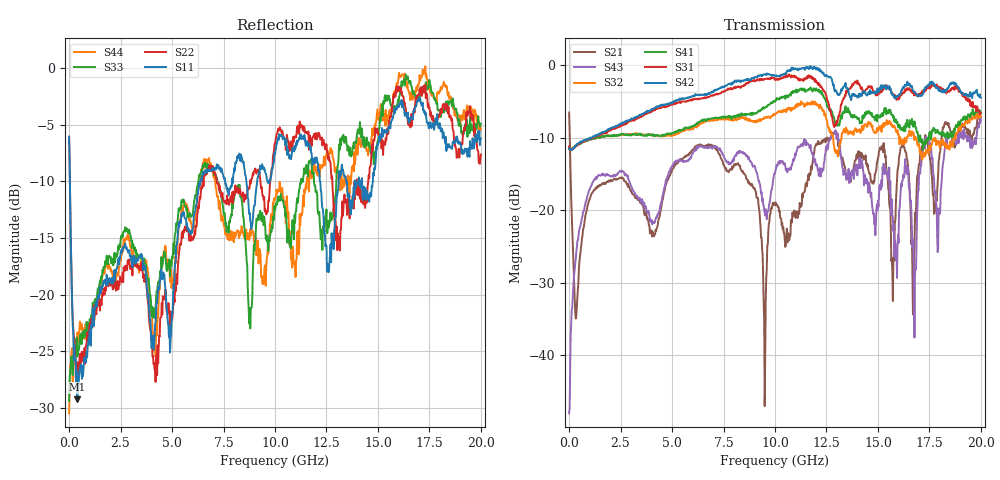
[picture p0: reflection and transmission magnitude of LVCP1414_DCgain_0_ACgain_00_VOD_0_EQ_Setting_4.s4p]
!Agilent Technologies,N5230A,MY46400459,A.07.50.48
!Agilent N5230A: A.07.50.48
!Date: Tuesday, April 17, 2012 18:34:43
!Correction: S11(Full 4 Port(1,2,3,4))
!S12(Full 4 Port(1,2,3,4))
!S13(Full 4 Port(1,2,3,4))
!S14(Full 4 Port(1,2,3,4))
!S21(Full 4 Port(1,2,3,4))
!S22(Full 4 Port(1,2,3,4))
!S23(Full 4 Port(1,2,3,4))
!S24(Full 4 Port(1,2,3,4))
!S31(Full 4 Port(1,2,3,4))
!S32(Full 4 Port(1,2,3,4))
!S33(Full 4 Port(1,2,3,4))
!S34(Full 4 Port(1,2,3,4))
!S41(Full 4 Port(1,2,3,4))
!S42(Full 4 Port(1,2,3,4))
!S43(Full 4 Port(1,2,3,4))
!S44(Full 4 Port(1,2,3,4))
!S4P File: Measurements: <S11,S12,S13,S14>,
!<S21,S22,S23,S24>,
!<S31,S32,S33,S34>,
!<S41,S42,S43,S44>:
# Hz S  dB  R 50
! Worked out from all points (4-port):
!   801 points, 300 kHz to 20 GHz, reference 50 ohm
!   strongest paths, dB at 300 kHz, 5 GHz, 10 GHz, 15 GHz, 20 GHz:
!     S42: -11.5, -5.1, -1.5, -3.4, -4.5
!     S31: -11.2, -5.4, -2.0, -4.1, -6.6
!     S41: -11.3, -9.3, -5.0, -7.0, -6.5
!     S32: -11.4, -9.7, -6.7, -9.0, -7.1
!     S43: -48.1, -13.9, -14.9, -18.7, -7.6
!     S21: -6.5, -14.4, -19.3, -12.8, -7.1
!   lowest |S11| = -29.2 dB at 400.3 MHz (marker M1), VSWR 1.07, Z = 53.2 + j1.51 ohm
!   |S11| at or under -10 dB: 37.55 MHz to 6.371 GHz (6.334 GHz wide, 198 % of centre); 8.609 GHz to 9.135 GHz (526.1 MHz wide, 5.93 % of centre); 12.19 GHz to 13.1 GHz (902.9 MHz wide, 7.14 % of centre)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
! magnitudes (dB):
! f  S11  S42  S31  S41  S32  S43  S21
! 300 kHz  -6.1  -11.5  -11.2  -11.3  -11.4  -48.1  -6.5
! 400.3 MHz  -29.2  -10.9  -10.9  -11.0  -10.9  -24.2  -32.3
! 10.1 GHz  -6.6  -1.4  -2.0  -4.5  -6.6  -13.9  -19.2
! 12.85 GHz  -16.0  -2.7  -8.3  -7.1  -10.9  -9.4  -9.3
! 14.03 GHz  -10.0  -4.4  -2.4  -7.4  -8.9  -13.8  -12.1
! 16.8 GHz  -3.5  -3.8  -3.9  -8.4  -9.9  -28.4  -20.3
! 20 GHz  -6.2  -4.5  -6.6  -6.5  -7.1  -7.6  -7.1
